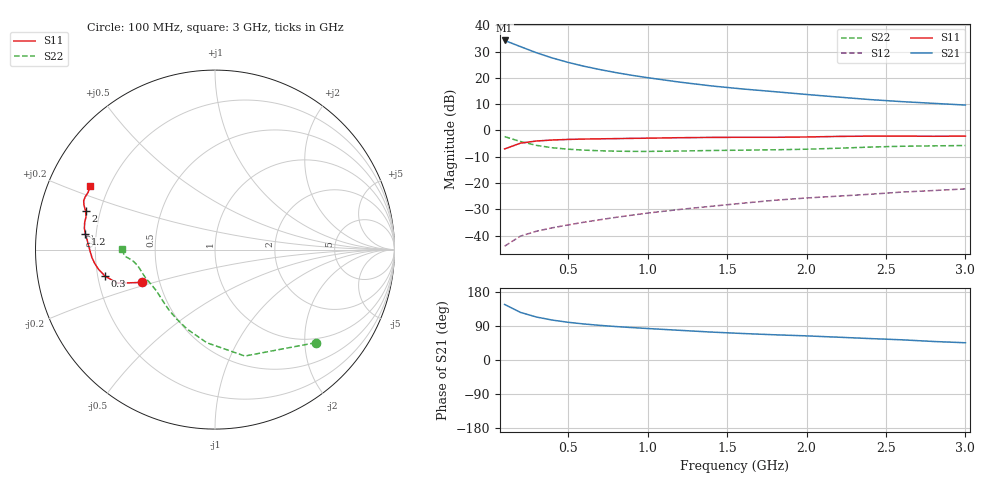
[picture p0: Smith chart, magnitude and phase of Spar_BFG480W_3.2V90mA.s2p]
! Filename: 3_290BFG480.001
! Title: BFG480W
! Bias: Vce=3.2V; Ic=90mA
! Company: NXP Semiconductors NL
! User: Quality&Reliability T&D
! Measure time: 10 Nov 1999 / 11:57:46
#  MHz  S  MA  R 50
! Freq  S11  S21  S12  S22  :
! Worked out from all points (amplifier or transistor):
!   20 points, 100 MHz to 3 GHz, reference 50 ohm
!   highest |S21| = 34.2 dB at 100 MHz (marker M1)
!   |S21| within 3 dB of that: start of sweep to 228.2 MHz
!   unconditionally stable (mu >= 1): 733.6 MHz to end of sweep
!   at 400 MHz: K = 0.80, MSG = 32.3 dB, |S12| = -37.0 dB
!   at 1.2 GHz: K = 1.07, MAG = 22.6 dB, |S12| = -30.0 dB
!   at 3 GHz: K = 1.05, MAG = 14.5 dB, |S12| = -22.2 dB
!   S11 on the Smith chart (normalised r, x): 100 MHz: 0.40, -0.18; 300 MHz: 0.23, -0.11; 1.2 GHz: 0.16, +0.06; 2 GHz: 0.14, +0.14; 3 GHz: 0.13, +0.24
100  0.4451 -155.8  51.41 146.6  0.006313 69.5  0.7641 -42.7
200  0.5737 -160.9  39.23 125.6  0.009817 60.5  0.6159 -74.3
300  0.6301 -166.4  30.05 113.4  0.01213 59.0  0.5209 -95.0
400  0.6586 -170.5  23.88 105.3  0.0141 60.6  0.4691 -109.4
500  0.6752 -173.6  19.68 99.5  0.01601 62.7  0.4402 -119.7
600  0.6866 -176.2  16.62 95.0  0.01802 64.5  0.4228 -127.4
700  0.6934 -178.4  14.37 91.4  0.02009 66.7  0.4112 -133.3
800  0.6997 179.6  12.6 88.3  0.02227 68.3  0.4039 -138.3
900  0.7072 177.7  11.2 85.6  0.02449 70.1  0.4003 -142.5
1000  0.7135 175.9  10.07 83.1  0.02686 71.1  0.3998 -146.3
1200  0.7282 173.0  8.313 78.4  0.03146 72.7  0.4063 -152.4
1400  0.7376 170.6  7.035 73.7  0.03614 73.7  0.416 -156.9
1600  0.7415 168.3  6.139 69.9  0.04144 74.5  0.422 -160.4
1800  0.7415 165.7  5.459 66.5  0.04713 75.0  0.4291 -164.1
2000  0.7518 163.4  4.832 63.6  0.05203 75.7  0.4401 -168.3
2200  0.7704 161.3  4.312 60.2  0.0564 75.6  0.4595 -171.9
2400  0.7805 159.6  3.863 56.5  0.06128 75.0  0.4829 -174.2
2600  0.7805 157.9  3.533 53.3  0.06738 74.3  0.501 -175.6
2800  0.7755 155.7  3.275 48.9  0.07211 72.9  0.5096 -177.4
3000  0.781 153.0  3.042 45.5  0.07746 72.1  0.517 179.7
